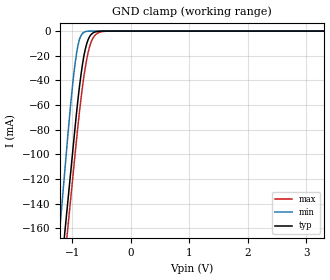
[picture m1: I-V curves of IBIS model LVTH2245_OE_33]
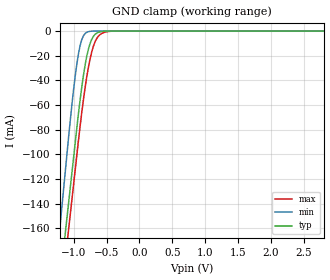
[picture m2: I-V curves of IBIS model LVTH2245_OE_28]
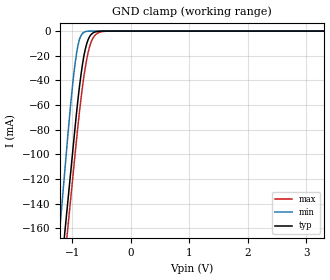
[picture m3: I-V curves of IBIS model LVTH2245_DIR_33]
| TEXAS INSTRUMENTS INCORPORATED
| Standard Linear and Logic Group
| IBIS Model of SN74LVTH2245
| 3.3-V ABT OCTAL BUS TRANSCEIVERS WITH 3-STATE OUTPUTS
| This file contains package information for the following:
|  SSOP 20-pin (DB) package as [Component] LVTH2245_DB
|  SOIC 20-pin (DW) package as [Component] LVTH2245_DW
|  TSSOP 20-pin (PW) package as [Component] LVTH2245_PW
| This device can be powered at the following Vccs:
|  3.3 volt Vcc
|  2.8 volt Vcc
| This file provides unique models under the [Model Selector] for each Vcc.
| For operation at a specific Vcc, select the appropriate model after each
| [Model Selector] keyword.
[IBIS Ver]   3.2
[Comment char]  |_char
[File Name]   sn74lvth2245.ibs
[File Rev]   1.1 | x_die
[Date]   June 18, 2002
[Source]   Data created from TI-SPICE simulations at TI-SLL.
[Notes]   The following is an IBIS list for the LVTH2245.
   Please contact sllibis@ti.com with questions and
   comments concerning SLL IBIS models.
   - Due to presence of BUS HOLD at input, GND-CLAMP curves
   have non-monotonic warnings.
   - Non-monotonic data in pullup as the device is
   overvoltage tolerant.
   - We omitted Power_Clamp table data from the input models,
   since there is no power clamp diode at input.
[Disclaimer] Property of Texas Instruments Incorporated.  Unauthorized
   reproduction and/or distribution is strictly prohibited.
   This product is protected under copyright law.
   Created  2002, (C) Copyright  2002, Texas Instruments
   Incorporated, All Rights Reserved
   UNLESS THERE IS A SIGNED, WRITTEN AGREEMENT TO THE
   CONTRARY, TEXAS INSTRUMENTS (TI) IS PROVIDING THE IBIS
   MODELS  AND WITHOUT ANY WARRANTY, EXPRESSED OR
   IMPLIED.  TI assumes no liability for:
   1) the accuracy of the IBIS models provided to your
   company;
   2) the proper functioning of these IBIS Models in your
   design or for any resulting applications; or
   3) infringement of patents, copyrights or intellectual
   property rights resulting from your use of these IBIS
   models.
   TI provides IBIS Models as a service to our customers.
   You and your company shall not distribute, sell or give
   these models to anyone else without prior written
   permission from TI.
   TI reserves the right to make changes to our products or
   to discontinue any semiconductor product or service
   without notice, and advises our customers to obtain the
   latest version of relevant information to verify, before
   placing orders, that the information being relied on is
   current.
   Please be aware that your receipt and use of the IBIS
   information provided shall serve as acceptance of these
   terms and conditions.  If you do not accept these terms,
   you should return or destroy the IBIS models and any
   other accompanying information immediately.
| Component LVTH2245_DB 20-pin SSOP
[Component]   LVTH2245_DB
[Manufacturer]   Texas Instruments, Inc.
[Package]
|   typ   min   max
R_pkg   4.000e-02   3.500e-02   5.100e-02
L_pkg   3.495e-09   3.035e-09   4.314e-09
C_pkg   4.200e-13   3.460e-13   5.020e-13
[Pin]   signal_name   model_name   R_pin   L_pin   C_pin
1   DIR   LVTH2245_DIR   4.900e-02   4.310e-09   5.020e-13
2   A1   LVTH2245_AIO   4.800e-02   3.903e-09   4.870e-13
3   A2   LVTH2245_AIO   3.500e-02   3.189e-09   3.960e-13
4   A3   LVTH2245_AIO   3.500e-02   3.036e-09   3.470e-13
5   A4   LVTH2245_AIO   3.500e-02   3.035e-09   3.670e-13
6   A5   LVTH2245_AIO   3.500e-02   3.035e-09   3.670e-13
7   A6   LVTH2245_AIO   3.500e-02   3.036e-09   3.470e-13
8   A7   LVTH2245_AIO   3.500e-02   3.189e-09   3.970e-13
9   A8   LVTH2245_AIO   4.700e-02   3.899e-09   4.880e-13
10   GND   GND   5.100e-02   4.314e-09   5.000e-13
11   B8   LVTH2245_BIO   5.100e-02   4.314e-09   5.000e-13
12   B7   LVTH2245_BIO   4.700e-02   3.899e-09   4.880e-13
13   B6   LVTH2245_BIO   3.500e-02   3.189e-09   3.970e-13
14   B5   LVTH2245_BIO   3.500e-02   3.036e-09   3.460e-13
15   B4   LVTH2245_BIO   3.500e-02   3.035e-09   3.670e-13
16   B3   LVTH2245_BIO   3.500e-02   3.035e-09   3.670e-13
17   B2   LVTH2245_BIO   3.500e-02   3.036e-09   3.460e-13
18   B1   LVTH2245_BIO   3.500e-02   3.189e-09   3.970e-13
19   NOE   LVTH2245_OE   4.700e-02   3.899e-09   4.880e-13
20   VCC   POWER   5.100e-02   4.314e-09   5.020e-13
| Component LVTH2245_DW 20-pin SOIC
[Component]   LVTH2245_DW
[Manufacturer]   Texas Instruments, Inc.
[Package]
|   typ   min   max
R_pkg   3.800e-02   3.300e-02   4.500e-02
L_pkg   5.012e-09   4.110e-09   6.349e-09
C_pkg   7.170e-13   5.300e-13   8.680e-13
[Pin]   signal_name   model_name   R_pin   L_pin   C_pin
1   DIR   LVTH2245_DIR   4.200e-02   6.336e-09   8.650e-13
2   A1   LVTH2245_AIO   4.300e-02   5.542e-09   8.670e-13
3   A2   LVTH2245_AIO   3.400e-02   4.714e-09   7.320e-13
4   A3   LVTH2245_AIO   3.400e-02   4.377e-09   5.910e-13
5   A4   LVTH2245_AIO   3.600e-02   4.130e-09   5.330e-13
6   A5   LVTH2245_AIO   3.500e-02   4.111e-09   5.300e-13
7   A6   LVTH2245_AIO   3.400e-02   4.284e-09   5.830e-13
8   A7   LVTH2245_AIO   3.400e-02   4.634e-09   7.260e-13
9   A8   LVTH2245_AIO   4.000e-02   5.518e-09   8.650e-13
10   GND   GND   4.300e-02   6.349e-09   8.660e-13
11   B8   LVTH2245_BIO   4.100e-02   6.281e-09   8.610e-13
12   B7   LVTH2245_BIO   4.500e-02   5.561e-09   8.680e-13
13   B6   LVTH2245_BIO   3.300e-02   4.778e-09   7.420e-13
14   B5   LVTH2245_BIO   3.500e-02   4.414e-09   5.960e-13
15   B4   LVTH2245_BIO   3.500e-02   4.110e-09   5.330e-13
16   B3   LVTH2245_BIO   3.600e-02   4.130e-09   5.330e-13
17   B2   LVTH2245_BIO   3.400e-02   4.377e-09   5.910e-13
18   B1   LVTH2245_BIO   3.400e-02   4.714e-09   7.310e-13
19   NOE   LVTH2245_OE   4.300e-02   5.569e-09   8.680e-13
20   VCC   POWER   4.200e-02   6.308e-09   8.640e-13
| Component LVTH2245_PW 20-pin TSSOP
[Component]   LVTH2245_PW
[Manufacturer]   Texas Instruments, Inc.
[Package]
|   typ   min   max
R_pkg   5.000e-02   4.200e-02   6.000e-02
L_pkg   2.802e-09   2.248e-09   3.553e-09
C_pkg   3.170e-13   2.020e-13   4.430e-13
[Pin]   signal_name   model_name   R_pin   L_pin   C_pin
1   DIR   LVTH2245_DIR   5.500e-02   3.461e-09   4.400e-13
2   A1   LVTH2245_AIO   5.500e-02   3.150e-09   4.010e-13
3   A2   LVTH2245_AIO   4.200e-02   2.619e-09   3.020e-13
4   A3   LVTH2245_AIO   4.500e-02   2.273e-09   2.020e-13
5   A4   LVTH2245_AIO   4.500e-02   2.248e-09   2.240e-13
6   A5   LVTH2245_AIO   4.500e-02   2.273e-09   2.260e-13
7   A6   LVTH2245_AIO   4.400e-02   2.323e-09   2.050e-13
8   A7   LVTH2245_AIO   4.600e-02   2.704e-09   3.070e-13
9   A8   LVTH2245_AIO   6.000e-02   3.265e-09   4.110e-13
10   GND   GND   5.700e-02   3.506e-09   4.360e-13
11   B8   LVTH2245_BIO   5.800e-02   3.553e-09   4.370e-13
12   B7   LVTH2245_BIO   5.800e-02   3.193e-09   4.050e-13
13   B6   LVTH2245_BIO   4.200e-02   2.704e-09   3.110e-13
14   B5   LVTH2245_BIO   4.600e-02   2.392e-09   2.100e-13
15   B4   LVTH2245_BIO   4.700e-02   2.334e-09   2.290e-13
16   B3   LVTH2245_BIO   4.700e-02   2.300e-09   2.270e-13
17   B2   LVTH2245_BIO   4.700e-02   2.349e-09   2.070e-13
18   B1   LVTH2245_BIO   4.500e-02   2.677e-09   3.060e-13
19   NOE   LVTH2245_OE   6.000e-02   3.235e-09   4.060e-13
20   VCC   POWER   5.600e-02   3.487e-09   4.430e-13
| Model LVTH2245_OE
[Model Selector]   LVTH2245_OE
LVTH2245_OE_33   3.3 volt Vcc
LVTH2245_OE_28   2.8 volt Vcc
| Model LVTH2245_DIR
[Model Selector]   LVTH2245_DIR
LVTH2245_DIR_33   3.3 volt Vcc
LVTH2245_DIR_28   2.8 volt Vcc
| Model LVTH2245_AIO
[Model Selector]   LVTH2245_AIO
LVTH2245_AIO_33   3.3 volt Vcc
LVTH2245_AIO_28   2.8 volt Vcc
| Model LVTH2245_BIO
[Model Selector]   LVTH2245_BIO
LVTH2245_BIO_33   3.3 volt Vcc
LVTH2245_BIO_28   2.8 volt Vcc
| Models and submodels in the file (8): LVTH2245_OE_33 (Input), LVTH2245_OE_28 (Input), LVTH2245_DIR_33 (Input), LVTH2245_DIR_28 (Input), LVTH2245_AIO_33 (I/O), LVTH2245_AIO_28 (I/O), LVTH2245_BIO_33 (I/O), LVTH2245_BIO_28 (I/O)
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[Model]   LVTH2245_OE_33
Model_type  Input
Vinl = 0.8
Vinh = 2.34
| variable   typ   min   max
C_comp   4.61pF   3.55pF   5.97pF
[Temperature Range]   40   -40   100
| Ambient temperature   25   -40   85
[Voltage range]   3.3   3   3.6
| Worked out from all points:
|   GND clamp passes 1 mA (typ) near -0.62 V on its own axis
[GND Clamp]
| LVTH2245_OE_33
|   Voltage   I(typ)   I(min)   I(max)
-5.5V     -2.407A    -2.649A    -2.406A
-1.22V    -209.3mA   -166mA     -230mA
-1.205V   -202mA     -157.6mA   -222.8mA
-1.125V   -163.1mA   -113mA     -184.2mA
-1.075V   -138.8mA   -85.25mA   -160.1mA
-975mV    -90.17mA   -36.12mA   -112mA
-900mV    -55.28mA   -11.44mA   -76.47mA
-825mV    -27.42mA   -1.98mA    -45.67mA
-775mV    -14.64mA   -464.8uA   -29.41mA
-650mV    -1.684mA   -2.076uA   -6.132mA
-395mV    -1.224uA   -43.32pA   -35.77uA
3.3V      16.15pA    8.657pA    1.272nA
[Model]   LVTH2245_OE_28
Model_type  Input
Vinl = 0.8
Vinh = 2.0
| variable   typ   min   max
C_comp   4.64pF   3.65pF   6.00pF
[Temperature Range]   40   -40   100
| Ambient temperature   25   -40   85
[Voltage range]   2.8   2.7   2.9
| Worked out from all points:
|   GND clamp passes 1 mA (typ) near -0.62 V on its own axis
[GND Clamp]
| LVTH2245_OE_28
|   Voltage   I(typ)   I(min)   I(max)
-5.5V     -2.407A    -2.649A    -2.406A
-1.22V    -209.3mA   -166mA     -230mA
-1.205V   -202mA     -157.6mA   -222.8mA
-1.125V   -163.1mA   -113mA     -184.2mA
-1.075V   -138.8mA   -85.25mA   -160.1mA
-975mV    -90.17mA   -36.12mA   -112mA
-900mV    -55.28mA   -11.44mA   -76.47mA
-800mV    -20.27mA   -984.6uA   -36.91mA
-675mV    -2.699mA   -6.758uA   -8.728mA
-575mV    -336.8uA   -57.38nA   -1.991mA
-425mV    -3.297uA   -110.8pA   -102.1uA
2.8V      13.7pA     7.338pA    757.3pA
[Model]   LVTH2245_DIR_33
Model_type  Input
Vinl = 0.8
Vinh = 2.34
| variable   typ   min   max
C_comp   4.62pF   3.56pF   5.96pF
[Temperature Range]   40   -40   100
| Ambient temperature   25   -40   85
[Voltage range]   3.3   3   3.6
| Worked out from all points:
|   GND clamp passes 1 mA (typ) near -0.62 V on its own axis
[GND Clamp]
| LVTH2245_DIR_33
|   Voltage   I(typ)   I(min)   I(max)
-5.5V     -2.407A    -2.649A    -2.406A
-1.22V    -209.3mA   -166mA     -230mA
-1.205V   -202mA     -157.6mA   -222.8mA
-1.125V   -163.1mA   -113mA     -184.2mA
-1.075V   -138.8mA   -85.25mA   -160.1mA
-975mV    -90.17mA   -36.12mA   -112mA
-900mV    -55.28mA   -11.44mA   -76.47mA
-825mV    -27.42mA   -1.98mA    -45.67mA
-775mV    -14.64mA   -464.8uA   -29.41mA
-650mV    -1.684mA   -2.076uA   -6.132mA
-395mV    -1.224uA   -43.32pA   -35.77uA
3.3V      16.15pA    8.657pA    1.272nA
